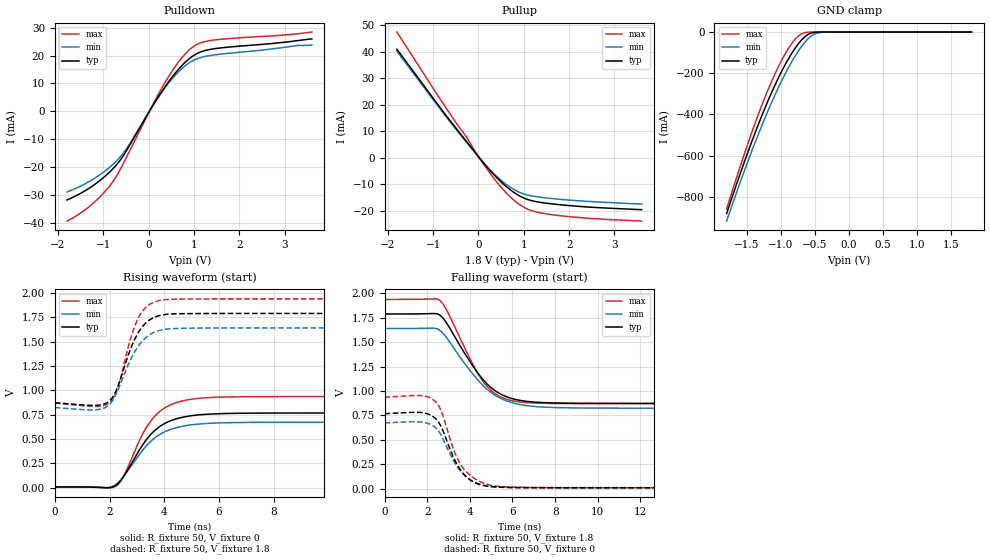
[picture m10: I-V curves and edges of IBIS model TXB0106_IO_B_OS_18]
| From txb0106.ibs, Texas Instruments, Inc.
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[Model]   TXB0106_IO_B_OS_18
Model_type  I/O
Vinl=0.5775
Vinh=1.2675
Enable   Active-High
Vref =   0
Rref =   1E6
Cref =   15p
Vmeas =   0.9
| variable   typ   min   max
C_comp   14.47pF   12.39pF   15.75pF
| C_pullup   15.26pF   12.17pF   17.22pF
| C_pulldown   15.30pF   13.57pF   16.01pF
| C_tri-state   14.47pF   12.39pF   15.75pF
[Temperature Range]   40   100   -40
| Ambient temperature   25   85   -40
[Voltage range]   1.8   1.65   1.95
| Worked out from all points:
|   slope of the pulldown table from 0 to 0.27 V, typ, clamps not added: 38.3 ohm
|   slope of the pullup table from 0 to 0.27 V, typ, clamps not added: 49.3 ohm
|   GND clamp passes 1 mA (typ) near -0.48 V on its own axis
|   rising waveform, R_fixture 50, V_fixture 0: 20-80 % time 1.16ns typ, 1.22ns min, 1.07ns max; typ from 0.009 V to 0.768 V
|   falling waveform, R_fixture 50, V_fixture 1.8: 20-80 % time 1.72ns typ, 1.85ns min, 1.53ns max; typ from 1.79 V to 0.873 V
|   rising waveform, R_fixture 50, V_fixture 1.8: 20-80 % time 757ps typ, 833ps min, 659ps max; typ from 0.873 V to 1.79 V
|   falling waveform, R_fixture 50, V_fixture 0: 20-80 % time 977ps typ, 1.06ns min, 1.01ns max; typ from 0.768 V to 0.009 V
[GND Clamp]
| TXB0104_IO_B_OS_18
|   Voltage   I(typ)   I(min)   I(max)
-1.8V     -881.6mA   -918mA     -859.1mA
-1.465V   -563.3mA   -608.7mA   -520.1mA
-1.315V   -433.3mA   -480.9mA   -383.5mA
-1.18V    -325.1mA   -373.3mA   -271.5mA
-1.05V    -230.3mA   -277.6mA   -175.9mA
-930mV    -152.7mA   -197.2mA   -100.9mA
-820mV    -91.61mA   -131.6mA   -46.23mA
-725mV    -48.5mA    -82.36mA   -14.2mA
-640mV    -20.26mA   -46.01mA   -2.365mA
-560mV    -5.64mA    -20.88mA   -230uA
-405mV    -139uA     -1.583mA   -687.7nA
1.8V      490pA      96.03nA    50.12pA
[Pulldown]
| TXB0104_IO_B_OS_18
|   Voltage   I(typ)   I(min)   I(max)
-1.8V     -31.63mA   -28.79mA   -39.16mA
-1.255V   -26.84mA   -24.53mA   -33.28mA
-1.01V    -23.83mA   -21.88mA   -29.47mA
-795mV    -20.59mA   -19.01mA   -25.24mA
-485mV    -13.88mA   -13.26mA   -16.22mA
80mV      1.766mA    1.752mA    2.073mA
355mV     8.684mA    8.321mA    10.19mA
675mV     15.37mA    14.42mA    18.03mA
955mV     19.58mA    17.97mA    22.83mA
1.15V     21.3mA     19.29mA    24.56mA
1.425V    22.37mA    20.16mA    25.51mA
3.6V      25.89mA    23.73mA    28.39mA
[Pullup]
| TXB0104_IO_B_OS_18
|   Voltage   I(typ)   I(min)   I(max)
-1.8V     40.87mA    40.11mA    47.34mA
-670mV    14.98mA    14.51mA    17.65mA
-255mV    5.951mA    5.655mA    7.547mA
60mV      -853.7uA   -849.9uA   -1.05mA
275mV     -5.144mA   -4.871mA   -6.252mA
480mV     -8.758mA   -8.183mA   -10.67mA
670mV     -11.61mA   -10.72mA   -14.19mA
850mV     -13.78mA   -12.54mA   -16.9mA
1.14V     -15.98mA   -14.23mA   -19.69mA
1.555V    -17.2mA    -15.21mA   -21.25mA
2.485V    -18.59mA   -16.47mA   -22.83mA
3.6V      -19.52mA   -17.41mA   -23.79mA
[Ramp]
| TXB0104_IO_B_OS_18
| variable   typ   min   max
dV/dt_r   0.46/1.16E-09   0.40/1.23E-09   0.56/1.07E-09
dV/dt_f   0.55/1.73E-09   0.49/1.86E-09   0.65/1.54E-09
R_load = 50
[Rising Waveform]
| TXB0104_IO_B_OS_18
R_fixture =   50
C_fixture =   0
L_fixture =   0
V_fixture =   0
V_fixture_min = 0
V_fixture_max = 0
|   Time   V(typ)   V(min)   V(max)
0s        8.643mV    7.492mV    9.18mV
1.875ns   739.3uV    1.117mV    1.342mV
2.225ns   24.05mV    33.26mV    14.78mV
2.53ns    122.6mV    124.2mV    128.5mV
3.27ns    465mV      405.4mV    583.1mV
3.69ns    597.5mV    519.6mV    745.5mV
3.995ns   657.4mV    571.9mV    816.5mV
4.345ns   699.8mV    609.7mV    865.1mV
5.355ns   750.8mV    656.6mV    920.6mV
39.92ns   767.8mV    673.3mV    936.5mV
[Falling Waveform]
| TXB0104_IO_B_OS_18
R_fixture =   50
C_fixture =   0
L_fixture =   0
V_fixture =   1.8
V_fixture_min = 1.65
V_fixture_max = 1.95
|   Time   V(typ)   V(min)   V(max)
0s        1.79V      1.641V     1.939V
2.255ns   1.794V     1.644V     1.944V
2.58ns    1.779V     1.624V     1.931V
2.9ns     1.7V       1.549V     1.834V
4.115ns   1.266V     1.181V     1.283V
4.69ns    1.099V     1.042V     1.08V
5.39ns    975.4mV    931.3mV    945.7mV
6.32ns    905.5mV    862.9mV    888.7mV
9.665ns   874mV      825.1mV    870.2mV
39.92ns   873mV      823.6mV    869.1mV
[Rising Waveform]
| TXB0104_IO_B_OS_18
R_fixture =   50
C_fixture =   0
L_fixture =   0
V_fixture =   1.8
V_fixture_min = 1.65
V_fixture_max = 1.95
|   Time   V(typ)   V(min)   V(max)
0s        872.9mV    823.1mV    869.1mV
1.495ns   846mV      801.1mV    835.5mV
2.03ns    900.7mV    865.4mV    881.9mV
2.17ns    956.6mV    922.4mV    936.8mV
2.3ns     1.037V     997.6mV    1.025V
2.775ns   1.43V      1.319V     1.537V
3.08ns    1.606V     1.464V     1.757V
3.455ns   1.722V     1.569V     1.881V
4.045ns   1.779V     1.627V     1.932V
39.92ns   1.79V      1.641V     1.939V
[Falling Waveform]
| TXB0104_IO_B_OS_18
R_fixture =   50
C_fixture =   0
L_fixture =   0
V_fixture =   0
V_fixture_min = 0
V_fixture_max = 0
|   Time   V(typ)   V(min)   V(max)
0s        767.8mV    673.3mV    936.5mV
1.68ns    780.2mV    682.6mV    954mV
2.32ns    730.8mV    637.1mV    903.8mV
2.495ns   692.6mV    601mV      863.7mV
2.645ns   638.1mV    551mV      801.8mV
3.255ns   309.7mV    278.1mV    390.1mV
3.655ns   164.3mV    156.7mV    220mV
4.31ns    53.27mV    56.28mV    91.59mV
5.26ns    16.18mV    15.91mV    24.05mV
39.92ns   8.643mV    7.491mV    9.18mV
